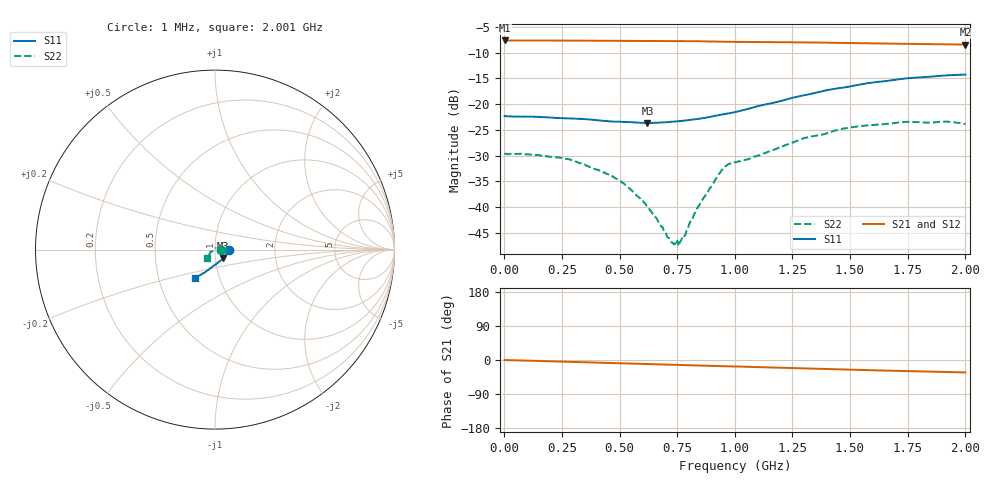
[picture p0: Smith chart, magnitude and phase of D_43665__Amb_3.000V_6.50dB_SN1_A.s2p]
! device id: 43665_
! dir: \\malibu\benchdata\1_engineers\tn_data\43665_75ohm\new\sparar\43665_\amb\3p000v\6p50db
! Serial: 1
! Insertion: A
! Temp: Amb
! VDD: 3.000V
! Attenuation Step: 6.50dB
! IDD: 1.455076e+00mA
! FILE NAME
! DATE 03-27-2009 08:34:58
! CORRECTED  DATA
#  Hz  S  RI  R  75
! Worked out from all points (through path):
!   401 points, 1 MHz to 2.001 GHz, reference 75 ohm
!   highest |S21| = -7.60 dB at 1 MHz (marker M1); lowest = -8.4 dB at 2.001 GHz (marker M2)
!   group delay of S21, straight-line fit = 46.6 ps
!   lowest |S11| = -23.7 dB at 621 MHz (marker M3), VSWR 1.14, Z = 81.9 - j7.63 ohm
!   |S11| at or under -10 dB: start of sweep to end of sweep
!   |S22| runs from -47.6 to -23.4 dB; largest |S21 - S12| = 0.0015
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1000000  0.0769 -0.00107  0.4169 -0.000627  0.4169 -0.000568  0.0333 -0.000342
2.36e8  0.0716 -0.0157  0.4147 -0.0285  0.4149 -0.0286  0.029 0.00829
3.36e8  0.0681 -0.0233  0.4132 -0.0408  0.4134 -0.0408  0.024 0.0112
4.61e8  0.06 -0.0323  0.4107 -0.056  0.4108 -0.0562  0.0173 0.011
5.06e8  0.0566 -0.0367  0.4094 -0.0616  0.4095 -0.0617  0.0144 0.0105
5.56e8  0.0526 -0.041  0.4076 -0.0677  0.4077 -0.0678  0.0103 0.0099
6.21e8  0.0462 -0.0464  0.4056 -0.0753  0.4056 -0.0754  0.00533 0.00854
6.71e8  0.0418 -0.0512  0.4041 -0.0814  0.4041 -0.0815  0.00288 0.00632
7.16e8  0.0372 -0.0558  0.4023 -0.087  0.4024 -0.087  0.000228 0.00495
7.36e8  0.0351 -0.0577  0.4016 -0.0895  0.4016 -0.0895  -0.00132 0.00411
7.66e8  0.032 -0.0606  0.4002 -0.0932  0.4003 -0.0932  -0.00363 0.00294
7.86e8  0.0299 -0.0626  0.3993 -0.0957  0.3992 -0.0958  -0.00516 0.00145
8.41e8  0.0232 -0.0681  0.3965 -0.1026  0.3963 -0.1026  -0.00953 -0.00333
9.31e8  0.0104 -0.0775  0.3898 -0.1129  0.39 -0.1127  -0.0178 -0.011
9.61e8  0.00718 -0.0802  0.388 -0.1151  0.3882 -0.1149  -0.0226 -0.0109
1.001e9  0.00217 -0.0836  0.3868 -0.1185  0.3869 -0.1184  -0.0252 -0.0104
1.056e9  -0.00646 -0.0894  0.3845 -0.1249  0.3848 -0.1248  -0.0253 -0.0142
1.336e9  -0.0455 -0.1183  0.3669 -0.1544  0.3674 -0.1545  -0.0345 -0.0345
1.501e9  -0.068 -0.1325  0.3547 -0.1696  0.3551 -0.1701  -0.0392 -0.0447
1.671e9  -0.0882 -0.1448  0.3425 -0.1836  0.3424 -0.1843  -0.0412 -0.0498
1.911e9  -0.1092 -0.1555  0.3253 -0.2006  0.325 -0.2007  -0.0439 -0.0514
2.001e9  -0.1138 -0.1568  0.3192 -0.2063  0.3179 -0.2072  -0.0424 -0.048
